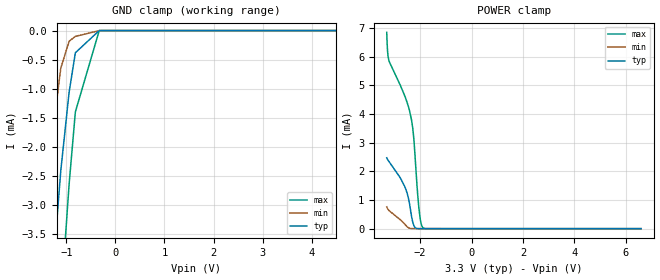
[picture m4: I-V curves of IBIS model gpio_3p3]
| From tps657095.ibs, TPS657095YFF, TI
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|   gpio_3p3 Model
[Model]   gpio_3p3
Model_type   Input
Vinl = 0.6
Vinh = 1.37
|   typ   min   max
|   (nom PVT)   (fast PVT)   (slow PVT)
C_comp   6.001e-13   5.500e-13   6.792e-13
| Where nom  PVT is Nominal Process, 3.3V, 27C
|   Fast PVT is Strong Process,  3.6V, -40C
|   Slow PVT is Weak Process,   3V, 125C
[Voltage Range]   3.3   3   3.6
|Junction Temperature
[Temperature Range]   27   125   -40
[Power Clamp Reference]   3.3   3   3.6
[GND Clamp Reference]   0   0   0
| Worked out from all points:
|   GND clamp passes 1 mA (typ) near -0.93 V on its own axis
|   POWER clamp passes 1 mA (typ) near -2.44 V on its own axis
[GND Clamp]
|   Voltage   I(typ)   I(min)   I(max)
-3.3V     -951.4mA   -747.3mA   -1.164A
-1.515V   -7.027mA   -3.734mA   -41.44mA
-1.435V   -5.98mA    -2.978mA   -17.42mA
-1.35V    -4.933mA   -2.232mA   -8.575mA
-1.113V   -2.405mA   -644.9uA   -4.697mA
-943.8mV  -1.06mA    -184.2uA   -2.641mA
-816mV    -380.9uA   -99.7uA    -1.396mA
-330mV    -261.4nA   -699.5nA   -365.8nA
6.6V      0A         0A         0A
[POWER Clamp]
|   Voltage   I(typ)   I(min)   I(max)
-3.3V     2.469mA    760.9uA    6.841mA
-3.268V   2.413mA    696.9uA    6.184mA
-3.217V   2.345mA    636.6uA    5.864mA
-2.581V   1.429mA    139.1uA    4.586mA
-2.452V   1.048mA    28.86uA    4.239mA
-2.339V   453.2uA    2.728uA    3.807mA
-2.245V   106.4uA    286.4nA    3.13mA
-2.122V   5.252uA    15.36nA    1.5mA
-2.049V   616.7nA    0A         724.8uA
-1.968V   42.67nA    0A         198.3uA
-1.885V   0A         0A         23.56uA
6.6V      0A         0A         0A
